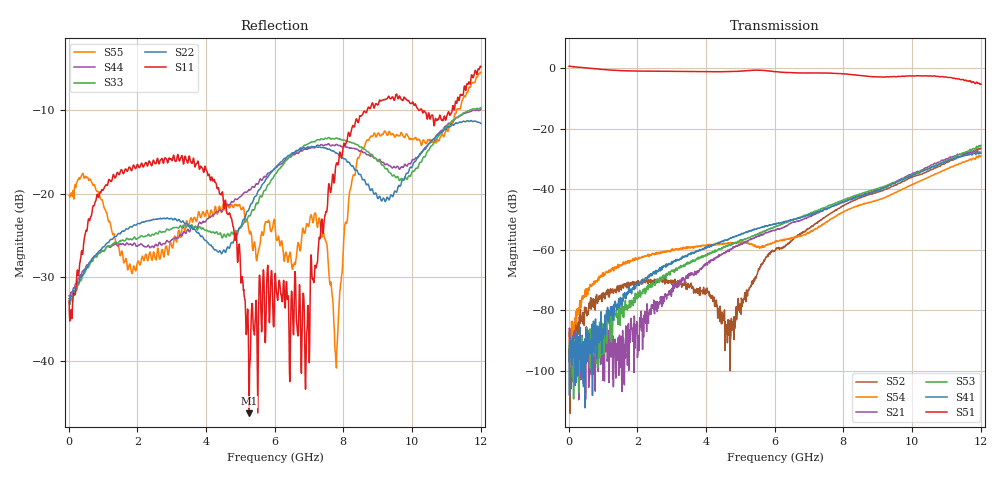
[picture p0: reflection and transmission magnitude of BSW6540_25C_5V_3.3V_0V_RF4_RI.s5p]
! Agilent Technologies	N5230C	MY49001333	A.09.33.09
!	Test time	=	2026-05-06 10:00
!	Product	=	BSW6540
!	Temp	=	25C
!	VDD	=	5
!	Control_High	=	3.3
!	Control_Low	=	0
!	Logic	=	RF4
!	Port1	=	RFC
!	Port2	=	RF1
!	Port3	=	RF2
!	Port4	=	RF3
!	Port5	=	RF4
!	V1	=	3.3 / 0
!	V2	=	3.3 / 0
!S5P File: Measurements: <S11,S12,S13,S14,S15>,
!<S21,S22,S23,S24,S25>,
!<S31,S32,S33,S34,S35>,
!<S41,S42,S43,S44,S45>,
!<S51,S52,S53,S54,S55>;
# HZ S RI R 50
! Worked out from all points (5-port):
!   1201 points, 10 MHz to 12.01 GHz, reference 50 ohm
!   strongest paths, dB at 10 MHz, 3.01 GHz, 6.01 GHz, 9.01 GHz, 12.01 GHz:
!     S51: 0.6, -1.1, -1.2, -2.9, -5.3
!     S41: -95.0, -63.9, -51.6, -40.4, -28.2
!     S53: -91.9, -67.1, -52.4, -39.8, -25.6
!     S21: -95.2, -73.0, -53.7, -40.1, -27.8
!     S54: -87.2, -59.7, -57.5, -43.7, -29.0
!     S52: -96.9, -70.3, -60.2, -41.0, -26.5
!   lowest |S11| = -46.3 dB at 5.25 GHz (marker M1), VSWR 1.01, Z = 50.4 + j0.238 ohm
!   |S11| at or under -10 dB: start of sweep to 8.698 GHz; 10.19346 GHz to 10.22896 GHz (35.5 MHz wide, 0.348 % of centre); 10.29 GHz to 11.17 GHz (880.4 MHz wide, 8.2 % of centre)
